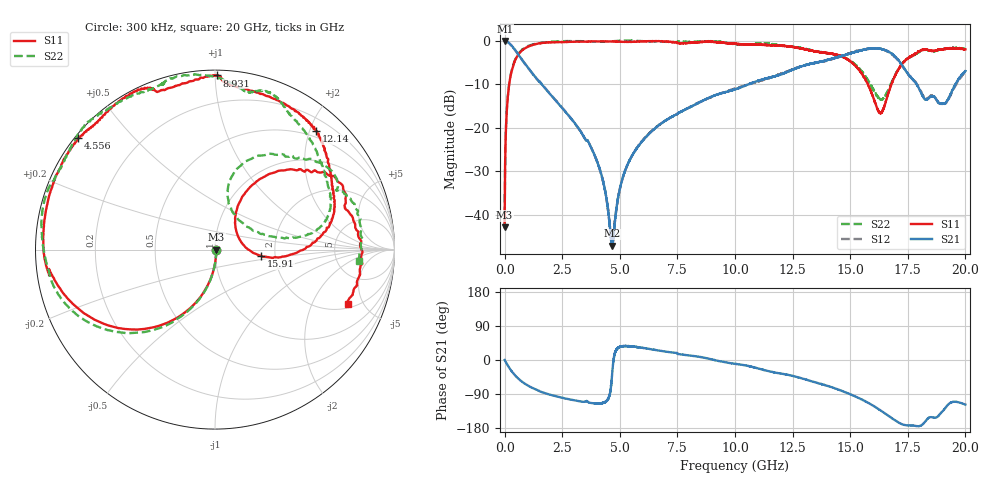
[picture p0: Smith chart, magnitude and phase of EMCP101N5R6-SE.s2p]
!EMCP101N5R6
!Johanson Technology Inc.
!www.johansontechnology.com
!Test Board Conditions:
!Substrate Type  RO4350B
!Substrate Thickness  10 mil
!Substrate Dk  3.66
!TL Type: GCPW
!TL Trace Width  20 mil
!TL Gap  10 mil
!PART MODE SINGLE ENDED (AKA BYPASS)
!DUT TOPOLOGY	SERIES-SHUNT
# MHz S  dB  R 50
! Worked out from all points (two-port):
!   20001 points, 300 kHz to 20 GHz, reference 50 ohm
!   highest |S21| = -0.06 dB at 4.3 MHz (marker M1); lowest = -47.1 dB at 4.664 GHz (marker M2)
!   |S21| within 3 dB of the highest: start of sweep to 578 MHz; 14.93 GHz to 16.82 GHz (1.89 GHz wide, 11.9 % of centre)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
!   lowest |S11| = -42.8 dB at 300 kHz (marker M3), VSWR 1.01, Z = 50.7 - j0.0843 ohm
!   |S11| at or under -10 dB: start of sweep to 200.4 MHz; 15.77 GHz to 16.79 GHz (1.024 GHz wide, 6.29 % of centre)
!   |S22| runs from -42.9 to 0.0 dB; largest |S21 - S12| = 0.022
!   S11 on the Smith chart (normalised r, x): 300 kHz: 1.01, -0.00; 4.556 GHz: 0.01, +0.36; 8.931 GHz: 0.03, +1.01; 12.14 GHz: 0.39, +2.10; 15.91 GHz: 1.69, -0.12; 20 GHz: 2.29, -3.76
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0.3  -42.82 -6.6  -0.08 -0.0  -0.06 0.0  -42.92 -5.7
4.3  -40.00 -46.1  -0.06 -0.4  -0.06 -0.5  -39.87 -46.8
168.297  -11.36 -106.6  -0.45 -17.3  -0.44 -17.3  -11.26 -106.5
525.292  -3.80 -136.6  -2.68 -45.1  -2.67 -45.3  -3.66 -134.9
1442.278  -0.67 -172.2  -9.05 -79.9  -9.05 -79.5  -0.65 -169.1
3334.25  -0.22 155.7  -21.10 -110.0  -21.13 -110.0  -0.13 158.6
4142.238  -0.16 144.7  -29.71 -114.3  -29.70 -114.5  -0.23 151.2
4556.232  -0.16 140.8  -42.06 -92.3  -41.91 -92.8  -0.17 146.2
4664.23  -0.17 139.8  -47.07 -37.2  -46.87 -39.5  -0.13 144.8
5301.22  -0.29 133.8  -28.84 36.8  -28.90 37.3  0.03 136.3
6667.2  -0.11 115.8  -19.52 25.2  -19.48 24.9  -0.20 120.4
8931.166  -0.26 89.3  -12.95 2.5  -13.05 2.4  -0.13 100.7
10000.15  -0.75 84.0  -11.18 -10.1  -10.99 -10.0  -0.83 80.7
12138.12  -1.22 49.6  -7.44 -37.4  -7.34 -37.2  -1.18 62.5
13334.1  -2.33 32.7  -5.26 -56.2  -5.25 -56.6  -2.20 41.9
14696.08  -3.74 11.7  -3.42 -82.8  -3.38 -82.5  -3.76 15.8
15907.06  -11.71 -7.6  -1.79 -117.4  -1.83 -117.9  -10.31 14.6
16309.06  -16.59 25.7  -1.88 -132.7  -1.87 -132.7  -13.40 43.2
16667.05  -11.89 61.3  -2.53 -147.6  -2.60 -147.9  -11.10 74.3
17642.03  -3.60 41.2  -8.50 -172.9  -8.44 -172.1  -3.69 52.1
18918.02  -2.03 11.0  -14.44 -141.3  -14.40 -142.3  -2.06 23.0
20000  -1.99 -22.3  -6.98 -117.7  -7.11 -115.2  -1.87 -4.7
